(* Logix 5000 AddOnInstructionDefinition export B256_COMPARE; software revision 30.00 *)

ADD_ON_INSTRUCTION B256_COMPARE   (* revision 1.0 20170916, vendor Kenneth A. Fischer *)
// Determines if C1<C2, C1=C2, or C1>C2
// Revision note:
// Rev1.0: 20170916 - Initial Release
VAR_IN_OUT
   Inp_C1 : DINT[22]; {required}
   Inp_C2 : DINT[22]; {required}
END_VAR
VAR_OUTPUT
   EQUAL : BOOL; {access Read Only}
   GREATER : BOOL; {access Read Only}
   LESS : BOOL; {access Read Only}
END_VAR
VAR
   C3 : DINT;
   i : DINT;
END_VAR

ROUTINE Logic   (* ladder *)
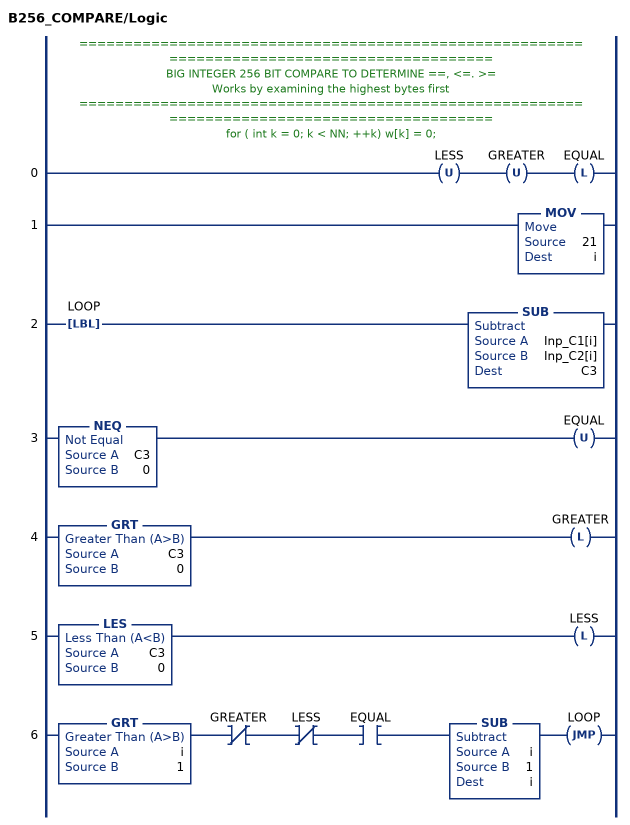
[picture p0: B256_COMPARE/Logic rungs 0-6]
   // ============================================================================================
   // BIG INTEGER 256 BIT COMPARE TO DETERMINE ==, <=. >=
   // Works by examining the highest bytes first
   // ============================================================================================
   // for ( int k = 0; k < NN; ++k) w[k] = 0;
   0: OTU(LESS)OTU(GREATER)OTL(EQUAL);
   1: MOV(21,i);
   2: LBL(LOOP)SUB(Inp_C1[i],Inp_C2[i],C3);
   3: NEQ(C3,0)OTU(EQUAL);
   4: GRT(C3,0)OTL(GREATER);
   5: LES(C3,0)OTL(LESS);
   6: GRT(i,1)XIO(GREATER)XIO(LESS)XIC(EQUAL)SUB(i,1,i)JMP(LOOP);
END_ROUTINE
END_ADD_ON_INSTRUCTION
